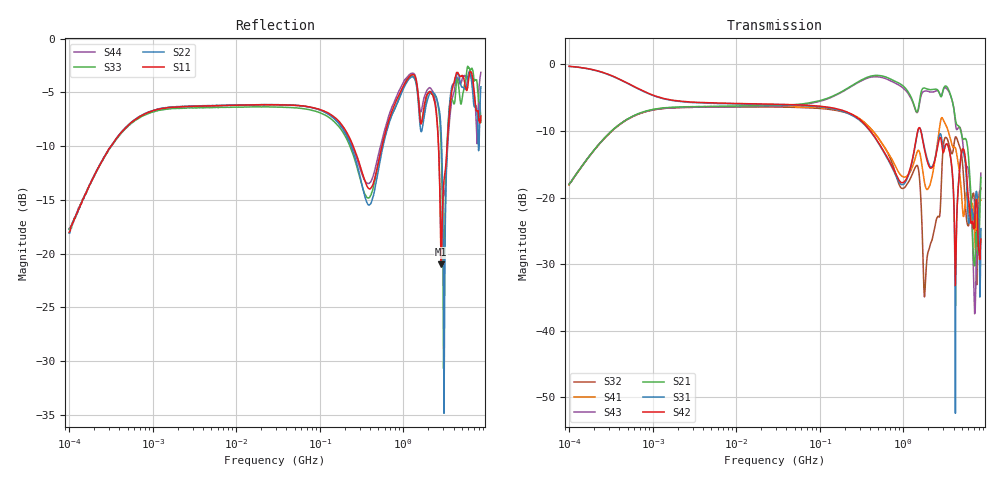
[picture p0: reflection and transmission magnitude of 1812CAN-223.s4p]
# Hz S dB R 50
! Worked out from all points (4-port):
!   801 points, 100 kHz to 8.5 GHz, reference 50 ohm
!   strongest paths, dB at 100 kHz, 1.721 MHz, 29.51 MHz, 502.3 MHz, 8.5 GHz:
!     S42: -0.3, -5.4, -6.0, -11.7, -26.2
!     S31: -0.3, -5.4, -6.1, -11.8, -24.7
!     S21: -18.1, -6.4, -6.2, -1.7, -17.0
!     S43: -18.0, -6.5, -6.3, -1.9, -16.3
!     S41: -18.1, -6.5, -6.3, -11.0, -20.4
!     S32: -18.0, -6.5, -6.4, -11.0, -18.6
!   lowest |S11| = -21.0 dB at 2.843 GHz (marker M1), VSWR 1.20, Z = 46.1 + j7.66 ohm
!   |S11| at or under -10 dB: start of sweep to 317.6 kHz; 251.5 MHz to 556.3 MHz (304.8 MHz wide, 75.5 % of centre); 2.64 GHz to 3.353 GHz (713 MHz wide, 23.8 % of centre)
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100000  -18.01 72.3  -18.06 74.8  -0.30 -7.1  -17.99 -105.9
        -18.06 74.8  -18.09 71.4  -18.06 -105.4  -0.30 -7.2
        -0.31 -7.0  -18.04 -105.5  -17.71 74.3  -17.99 74.3
        -18.10 -105.2  -0.26 -7.2  -17.95 73.9  -17.71 74.3
1.851923e9  -5.61 75.4  -3.60 -10.1  -13.24 61.1  -18.45 -167.8
            -3.60 -10.1  -6.43 80.9  -32.39 100.1  -13.58 60.1
            -13.24 61.1  -32.22 100.4  -5.95 80.9  -3.98 -12.5
            -18.43 -167.8  -13.56 60.0  -3.99 -12.4  -5.10 71.1
2.843154e9  -20.98 112.5  -4.86 -21.5  -10.67 27.8  -8.14 75.9
            -4.87 -21.6  -8.76 65.9  -18.57 103.9  -11.31 27.3
            -10.68 27.8  -18.65 103.7  -10.15 71.3  -4.80 -27.3
            -8.15 75.9  -11.31 27.3  -4.79 -27.2  -18.55 102.2
4.209908e9  -3.57 -127.5  -8.24 -56.7  -51.99 53.4  -12.52 -36.5
            -8.21 -56.7  -3.89 -131.4  -10.89 -14.9  -33.22 -0.2
            -52.38 42.4  -10.89 -14.9  -5.29 -131.1  -8.76 -71.4
            -12.52 -36.5  -33.20 1.2  -8.74 -71.1  -4.20 -126.9
5.385872e9  -3.95 -80.3  -11.19 -51.6  -13.76 -9.7  -22.31 125.9
            -11.18 -51.7  -4.65 -76.1  -18.58 -158.4  -13.05 -12.9
            -13.77 -9.9  -18.60 -158.1  -4.34 -60.2  -13.79 -80.6
            -22.27 125.7  -13.09 -12.7  -13.77 -80.1  -3.52 -79.0
7.256907e9  -5.85 27.2  -28.88 5.7  -20.87 22.6  -27.36 1.2
            -28.72 5.3  -6.34 29.3  -22.92 -16.8  -21.83 2.9
            -20.93 22.1  -22.85 -17.0  -3.88 31.7  -36.87 143.0
            -27.30 2.6  -21.82 2.8  -37.23 145.8  -6.09 18.0
8.5e9  -7.21 135.1  -16.97 67.8  -24.67 70.3  -20.47 25.9
       -16.96 67.7  -4.49 132.7  -18.55 36.7  -26.24 2.5
       -24.65 70.0  -18.59 36.0  -7.79 119.1  -16.27 74.2
       -20.41 25.5  -26.22 2.5  -16.32 74.7  -3.15 128.3
